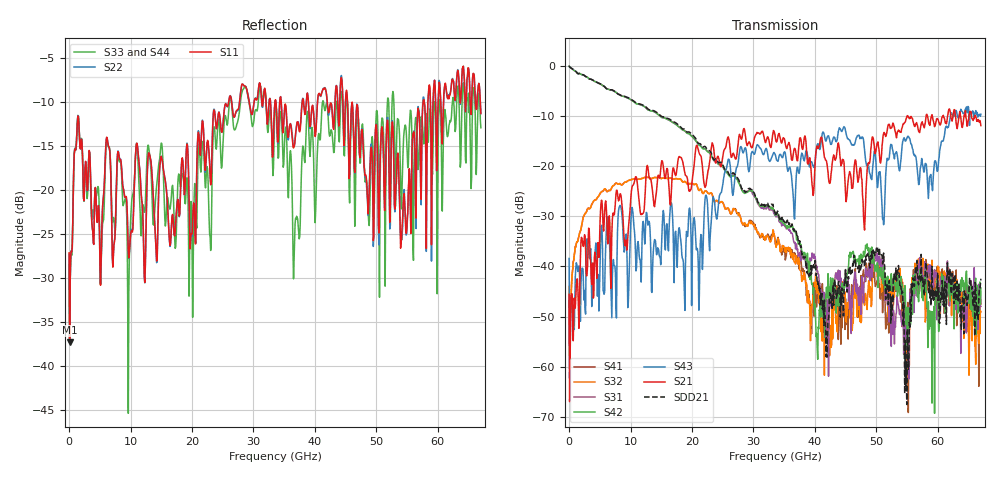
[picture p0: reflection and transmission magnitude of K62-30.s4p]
!Agilent Technologies,N5247A,US50470101,A.10.25.02
!Agilent N5247A: A.10.25.02
!Date: Tuesday, May 12, 2015 13:41:46
!Correction: Sdd11(Full 4 Port(1,2,3,4))
!Sdc11(Full 4 Port(1,2,3,4))
!Sdd12(Full 4 Port(1,2,3,4))
!Sdc12(Full 4 Port(1,2,3,4))
!Scd11(Full 4 Port(1,2,3,4))
!Scc11(Full 4 Port(1,2,3,4))
!Scd12(Full 4 Port(1,2,3,4))
!Scc12(Full 4 Port(1,2,3,4))
!Sdd21(Full 4 Port(1,2,3,4))
!Sdc21(Full 4 Port(1,2,3,4))
!Sdd22(Full 4 Port(1,2,3,4))
!Sdc22(Full 4 Port(1,2,3,4))
!Scd21(Full 4 Port(1,2,3,4))
!Scc21(Full 4 Port(1,2,3,4))
!Scd22(Full 4 Port(1,2,3,4))
!Scc22(Full 4 Port(1,2,3,4))
!Balanced Topology: BBAL
!S4P File: Measurements: <Sdd11,Sdc11,Sdd12,Sdc12>,
!<Scd11,Scc11,Scd12,Scc12>,
!<Sdd21,Sdc21,Sdd22,Sdc22>,
!<Scd21,Scc21,Scd22,Scc22>:
# Hz S  dB  R 50
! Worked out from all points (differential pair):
!   801 points, 10 MHz to 67 GHz, reference 50 ohm
!   strongest paths, dB at 10 MHz, 16.76 GHz, 33.51 GHz, 50.25 GHz, 67 GHz:
!     S21: -45.6, -22.2, -13.8, -15.2, -11.9
!     S43: -38.4, -28.2, -17.6, -23.7, -9.6
!     S42: 0.0, -11.2, -29.2, -44.2, -44.3
!     S31: 0.0, -11.2, -29.6, -38.9, -48.0
!     S32: -44.0, -22.5, -34.6, -39.6, -49.0
!     S41: -46.9, -22.5, -34.9, -41.8, -47.5
!   taken as a pair (ports 2,1 in; 4,3 out), SDD21 dB: 0.0, -11.0, -29.1, -37.0, -42.5
!   lowest |S11| = -37.4 dB at 93.74 MHz (marker M1), VSWR 1.03, Z = 48.8 - j0.477 ohm
!   |S11| at or under -10 dB: start of sweep to 25.98 GHz; 34.51 GHz to 37.94 GHz (3.427 GHz wide, 9.46 % of centre); 45.3 GHz to 57.61 GHz (12.31 GHz wide, 23.9 % of centre)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
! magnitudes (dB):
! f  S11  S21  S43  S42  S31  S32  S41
! 10 MHz  -27.2  -45.6  -38.4  0.0  0.0  -44.0  -46.9
! 93.74 MHz  -37.4  -67.0  -62.3  -0.2  -0.2  -57.9  -55.7
! 1.35 GHz  -12.4  -42.5  -40.2  -1.4  -1.4  -35.1  -35.0
! 14.33 GHz  -28.0  -23.5  -37.2  -9.5  -9.5  -22.2  -22.2
! 36.44 GHz  -15.1  -17.9  -25.4  -32.1  -34.3  -38.6  -38.4
! 40.29 GHz  -11.7  -16.2  -16.0  -53.4  -39.9  -43.6  -48.1
! 67 GHz  -11.4  -11.9  -9.6  -44.3  -48.0  -49.0  -47.5
